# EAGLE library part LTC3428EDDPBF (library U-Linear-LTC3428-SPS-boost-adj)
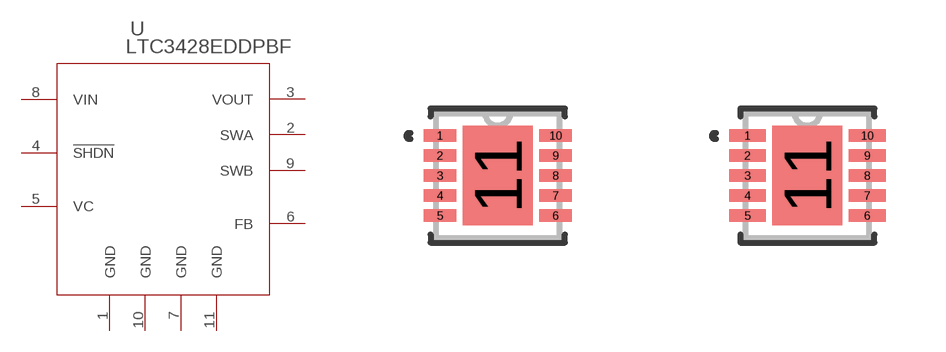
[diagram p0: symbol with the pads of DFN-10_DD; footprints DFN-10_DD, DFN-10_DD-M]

Designator prefix U

## LTC3428EDDPBF (MFR: Linear Technology; MPN: LTC3428EDD#PBF)  [DFN-10_DD]
1  GND  pwr
2  SWA  pas
3  VOUT  out
4  !SHDN  pas
5  VC  out
6  FB  pas
7  GND  pwr
8  VIN  in
9  SWB  pas
10  GND  pwr
11  GND  pas

## LTC3428EDDPBFDFN-10_DD-M (MANUFACTURER_PART_NUMBER: LTC3428EDD#PBF; VENDOR: Linear Technology)  [DFN-10_DD-M]
Pads as for DFN-10_DD

## LTC3428EDDPBFDFN-10_DD-L (MANUFACTURER_PART_NUMBER: LTC3428EDD#PBF; VENDOR: Linear Technology)  [DFN-10_DD-L]
Pads as for DFN-10_DD

## Footprint DFN-10_DD (pad centres in mm)
smd 0.813 x 0.305: 1 -1.448,1; 2 -1.448,0.5; 3 -1.448,0; 4 -1.448,-0.5; 5 -1.448,-1; 6 1.448,-1; 7 1.448,-0.5; 8 1.448,0; 9 1.448,0.5; 10 1.448,1
smd 1.753 x 2.489: 11 0,0

## Footprint DFN-10_DD-M (pad centres in mm)
smd 0.914 x 0.305: 1 -1.499,1; 2 -1.499,0.5; 3 -1.499,0; 4 -1.499,-0.5; 5 -1.499,-1; 6 1.499,-1; 7 1.499,-0.5; 8 1.499,0; 9 1.499,0.5; 10 1.499,1
smd 1.753 x 2.489: 11 0,0

## Footprint DFN-10_DD-L (pad centres in mm)
smd 0.711 x 0.305: 1 -1.397,1; 2 -1.397,0.5; 3 -1.397,0; 4 -1.397,-0.5; 5 -1.397,-1; 6 1.397,-1; 7 1.397,-0.5; 8 1.397,0; 9 1.397,0.5; 10 1.397,1
smd 1.753 x 2.489: 11 0,0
